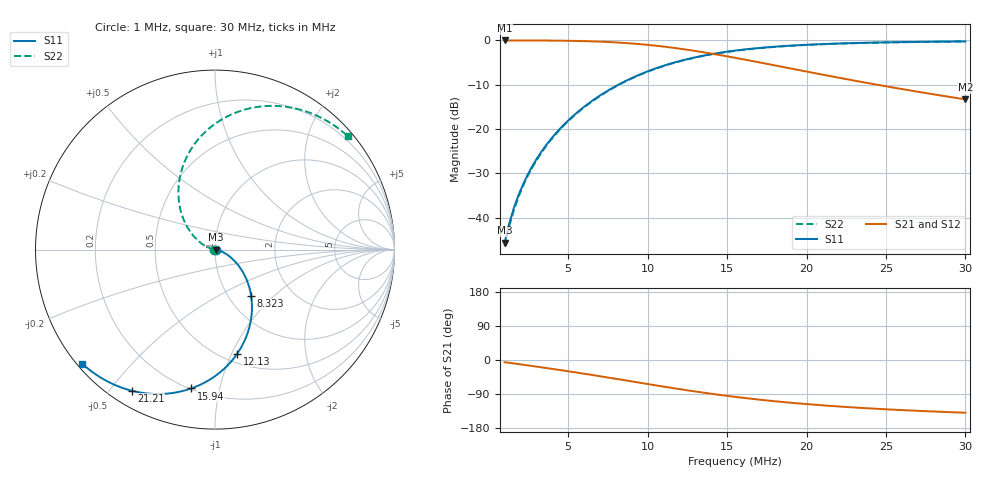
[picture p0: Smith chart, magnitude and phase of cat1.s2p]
# MHz S RI R 50
!SimSmith 16.9av
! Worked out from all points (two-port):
!   100 points, 1 MHz to 30 MHz, reference 50 ohm
!   highest |S21| = 0.00 dB at 1 MHz (marker M1); lowest = -13.3 dB at 30 MHz (marker M2)
!   |S21| within 3 dB of the highest: start of sweep to 14.07 MHz
!   lowest |S11| = -45.6 dB at 1 MHz (marker M3), VSWR 1.01, Z = 50.5 - j0.0553 ohm
!   |S11| at or under -10 dB: start of sweep to 8.154 MHz
!   |S22| runs from -46.4 to -0.2 dB; largest |S21 - S12| = 0
!   S11 on the Smith chart (normalised r, x): 1 MHz: 1.01, -0.00; 8.323 MHz: 1.27, -0.74; 12.13 MHz: 0.59, -1.05; 15.94 MHz: 0.20, -0.82; 21.21 MHz: 0.06, -0.57; 30 MHz: 0.01, -0.37
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1  0.00519 -0.000547  0.9947 -0.1  0.9947 -0.1  -0.00475 0.000508
1.292929  0.00857 -0.00116  0.9912 -0.1292  0.9912 -0.1292  -0.00799 0.00109
1.585859  0.0128 -0.00211  0.9868 -0.1585  0.9868 -0.1585  -0.012 0.00201
1.878788  0.0177 -0.00348  0.9815 -0.1877  0.9815 -0.1877  -0.0169 0.00333
2.171717  0.0234 -0.00534  0.9753 -0.2169  0.9753 -0.2169  -0.0225 0.00514
2.757576  0.037 -0.0108  0.9598 -0.2751  0.9598 -0.2751  -0.0358 0.0105
3.343434  0.0532 -0.0191  0.9403 -0.333  0.9403 -0.333  -0.0517 0.0187
4.222222  0.0811 -0.0381  0.9026 -0.4183  0.9026 -0.4183  -0.0794 0.0373
5.979798  0.1425 -0.1049  0.7944 -0.5782  0.7944 -0.5782  -0.1404 0.1034
7.151515  0.1785 -0.1732  0.6972 -0.6695  0.6972 -0.6695  -0.1762 0.1711
8.323232  0.2014 -0.2591  0.5824 -0.7408  0.5824 -0.7408  -0.1992 0.2563
9.494949  0.2045 -0.3572  0.4558 -0.7862  0.4558 -0.7862  -0.2025 0.3539
10.66667  0.1836 -0.4595  0.3256 -0.8026  0.3256 -0.8026  -0.1819 0.4557
12.13131  0.1241 -0.5795  0.1722 -0.7837  0.1722 -0.7837  -0.1231 0.5753
13.88889  0.0158 -0.6936  0.0202 -0.7167  0.0202 -0.7167  -0.0156 0.6891
15.64646  -0.1113 -0.7656  -0.0873 -0.6242  -0.0873 -0.6242  0.1108 0.7612
15.93939  -0.1328 -0.7737  -0.101 -0.6079  -0.101 -0.6079  0.1322 0.7693
17.9899  -0.2773 -0.8032  -0.1683 -0.4961  -0.1683 -0.4961  0.276 0.7992
20.62626  -0.4343 -0.7929  -0.2017 -0.373  -0.2017 -0.373  0.4325 0.7894
21.21212  -0.4641 -0.7861  -0.2039 -0.3498  -0.2039 -0.3498  0.4622 0.7827
25.31313  -0.6266 -0.7191  -0.194 -0.2251  -0.194 -0.2251  0.6244 0.7165
30  -0.7409 -0.6347  -0.1636 -0.1417  -0.1636 -0.1417  0.7387 0.6328
